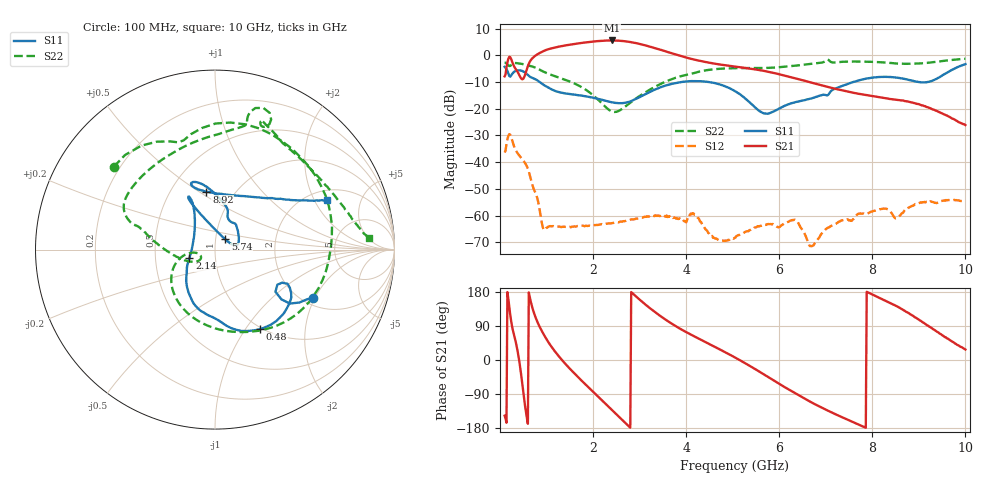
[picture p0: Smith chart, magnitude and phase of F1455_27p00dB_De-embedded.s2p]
! Integrated Device Technology
! Corporate Headquarters
! 6024 Silver Creek Valley Road
! San Jose, CA 95138  USA
! Phone:  1-408-284-8200
! Toll Free:  1-800-223-1366
! Webpage:  http://www.idt.com/
! Timing and RF Division
! 515 Groton Road, Suite 102
! Westford, MA 01886-6024
! Device:  F1455
! Description: 6-bit 0.5 dB Transmit Variable Gain Amplifier
! Frequency:  1400.0 -  2300.00 MHz
! Package:  6x6 mm Thin QFN Plastic Package: 28 pin
! State:  54
! Atten State:  27.0 dB
! Voltage:  +5.00 Volts
! Current:  217.622 mA
! Data:  The device was measured on a the F1455 evaluation board which has
!  individual transmission lines to the RF pins.  Data was collected
!  using a calibrated network analyzer.  The evaluation board was
!  de-embedded using a TRL calibration technique.
!  The reference plane is the edge of the package pin.
!  Pin  1 = CSb
!  Pin  2 = DATA
!  Pin  3 = CLK
!  Pin  4 = RSET
!  Pin  5 = GND
!  Pin  6 = RFIN  = Port 1
!  Pin  7 = GND
!  Pin  8 = NC
!  Pin  9 = NC
!  Pin 10 = NC
!  Pin 11 = NC
!  Pin 12 = NC
!  Pin 13 = NC
!  Pin 14 = /STBY
!  Pin 15 = GND
!  Pin 16 = RFOUT  = Port 2
!  Pin 17 = GND
!  Pin 18 = NC
!  Pin 19 = NC
!  Pin 20 = NC
!  Pin 21 = GND
!  Pin 22 = NC
!  Pin 23 = GND
!  Pin 24 = NC
!  Pin 25 = NC
!  Pin 26 = NC
!  Pin 27 = GND
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# GHz S dB R 50
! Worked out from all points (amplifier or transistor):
!   496 points, 100 MHz to 10 GHz, reference 50 ohm
!   highest |S21| = 5.6 dB at 2.4 GHz (marker M1)
!   |S21| within 3 dB of that: 1.099 GHz to 3.358 GHz (2.259 GHz wide, 101 % of centre)
!   unconditionally stable (mu >= 1): start of sweep to end of sweep
!   at 1.74 GHz: K = 413.11, MAG = 5.1 dB, |S12| = -63.8 dB
!   at 5.06 GHz: K = 1347.50, MAG = -2.3 dB, |S12| = -68.3 dB
!   at 10 GHz: K = 731.96, MAG = -17.4 dB, |S12| = -54.6 dB
!   S11 on the Smith chart (normalised r, x): 100 MHz: 2.27, -1.94; 480 MHz: 0.97, -1.17; 2.14 GHz: 0.75, -0.07; 5.74 GHz: 1.11, +0.13; 8.92 GHz: 0.74, +0.54; 10 GHz: 2.44, +2.56
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0.1  -4.29 -26.1  -7.86 -147.1  -36.39 47.5  -2.75 140.7
0.18  -6.70 -36.9  -1.28 161.2  -30.14 -6.4  -3.71 112.4
0.26  -6.99 -25.2  -2.27 88.9  -31.64 -77.2  -3.33 96.1
0.38  -5.64 -42.6  -6.22 23.0  -36.69 -118.9  -2.97 58.1
0.48  -5.85 -60.7  -8.98 -63.1  -38.93 -150.6  -3.23 31.3
0.66  -8.17 -88.1  -1.85 155.1  -46.20 140.4  -4.02 -11.2
0.78  -9.11 -103.1  0.11 107.8  -52.24 117.1  -4.72 -38.1
0.94  -11.05 -121.8  1.64 67.5  -65.35 120.1  -6.15 -68.6
1.32  -13.98 -141.8  3.45 1.8  -64.33 116.6  -8.64 -119.6
1.76  -15.07 -151.2  4.66 -55.2  -63.79 84.9  -11.96 -156.5
2.14  -16.42 -161.2  5.40 -100.3  -63.38 70.6  -17.11 -172.4
2.4  -17.53 -175.6  5.58 -131.3  -62.81 64.3  -20.97 -161.4
2.82  -17.11 146.5  4.93 179.2  -61.45 54.9  -17.49 -149.7
3.4  -12.31 118.5  2.35 120.2  -59.96 32.4  -11.17 -179.8
4.08  -9.68 116.1  -1.19 68.5  -59.68 17.7  -7.01 163.2
5.06  -13.49 112.0  -4.23 6.0  -68.28 34.8  -4.79 147.9
5.74  -21.87 45.3  -6.04 -43.3  -63.25 29.3  -4.70 119.8
6.36  -17.47 14.8  -8.64 -89.1  -61.74 -22.2  -3.85 88.6
6.7  -16.10 34.3  -10.25 -112.3  -71.45 -160.3  -3.16 78.4
8.36  -8.07 109.5  -16.29 151.7  -58.02 65.8  -2.79 62.3
8.92  -9.72 98.4  -17.97 112.4  -55.70 82.8  -3.13 39.8
10  -3.29 24.0  -26.10 27.6  -54.59 15.2  -1.28 4.5
